(* Logix 5000 AddOnInstructionDefinition export Banner_S15C_UI_PD_v2; software revision 32.00 *)

TYPE Banner_S15C_UI_PDI_v2 :   // UDT with all of the variables needed to control an IO-Link S15C MU or S15C MI.
STRUCT
   Data_Set_0 : Banner_S15C_UI_Set_0;   // English Data Set
   Data_Set_1 : Banner_S15C_UI_Set_1;   // Metric Data Set
   DTI : SINT[32];   // Array with Raw Process data being transferred into AOI.
END_STRUCT
END_TYPE

TYPE Banner_S15C_UI_Set_0 :
STRUCT
   Measurement_Value : DINT;
END_STRUCT
END_TYPE

TYPE Banner_S15C_UI_Set_1 :
STRUCT
   Measurement_Value : DINT;   // Current or Voltage values
   Measurement_Scale : INT;   // 250 = microAmps, 253 = microVolts
END_STRUCT
END_TYPE

ADD_ON_INSTRUCTION Banner_S15C_UI_PD_v2   (* revision 2.0, vendor Banner Engineering *)
// AOI that used with the S15C UI sensor.
VAR_IN_OUT
   Process_Data : Banner_S15C_UI_PDI_v2; {required}
END_VAR
VAR_INPUT
   Byte_Swap : BOOL; {required}
   Data_Set : SINT; {required}
END_VAR
VAR
   Temp : SINT[4]; {access None}
END_VAR

ROUTINE Logic   (* ladder *)
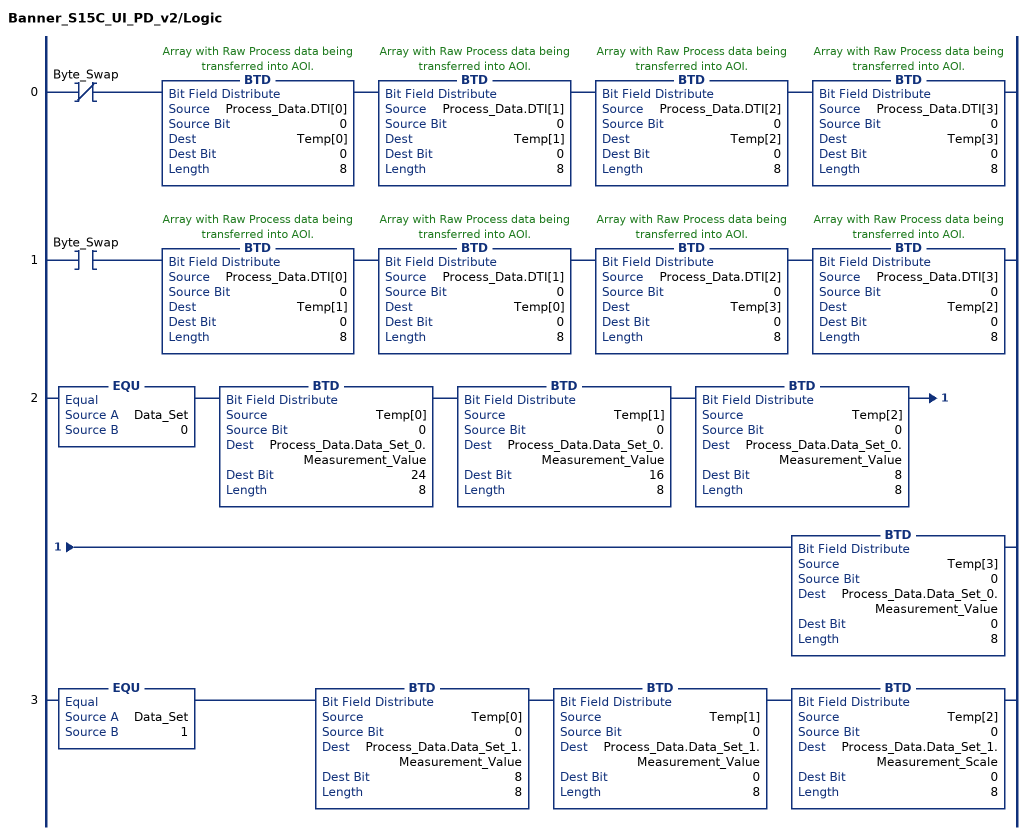
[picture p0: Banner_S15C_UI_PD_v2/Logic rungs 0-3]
   0: XIO(Byte_Swap)BTD(Process_Data.DTI[0],0,Temp[0],0,8)BTD(Process_Data.DTI[1],0,Temp[1],0,8)BTD(Process_Data.DTI[2],0,Temp[2],0,8)BTD(Process_Data.DTI[3],0,Temp[3],0,8);
   1: XIC(Byte_Swap)BTD(Process_Data.DTI[0],0,Temp[1],0,8)BTD(Process_Data.DTI[1],0,Temp[0],0,8)BTD(Process_Data.DTI[2],0,Temp[3],0,8)BTD(Process_Data.DTI[3],0,Temp[2],0,8);
   2: EQU(Data_Set,0)BTD(Temp[0],0,Process_Data.Data_Set_0.Measurement_Value,24,8)BTD(Temp[1],0,Process_Data.Data_Set_0.Measurement_Value,16,8)BTD(Temp[2],0,Process_Data.Data_Set_0.Measurement_Value,8,8)BTD(Temp[3],0,Process_Data.Data_Set_0.Measurement_Value,0,8);
   3: EQU(Data_Set,1)BTD(Temp[0],0,Process_Data.Data_Set_1.Measurement_Value,8,8)BTD(Temp[1],0,Process_Data.Data_Set_1.Measurement_Value,0,8)BTD(Temp[2],0,Process_Data.Data_Set_1.Measurement_Scale,0,8);
END_ROUTINE
END_ADD_ON_INSTRUCTION
